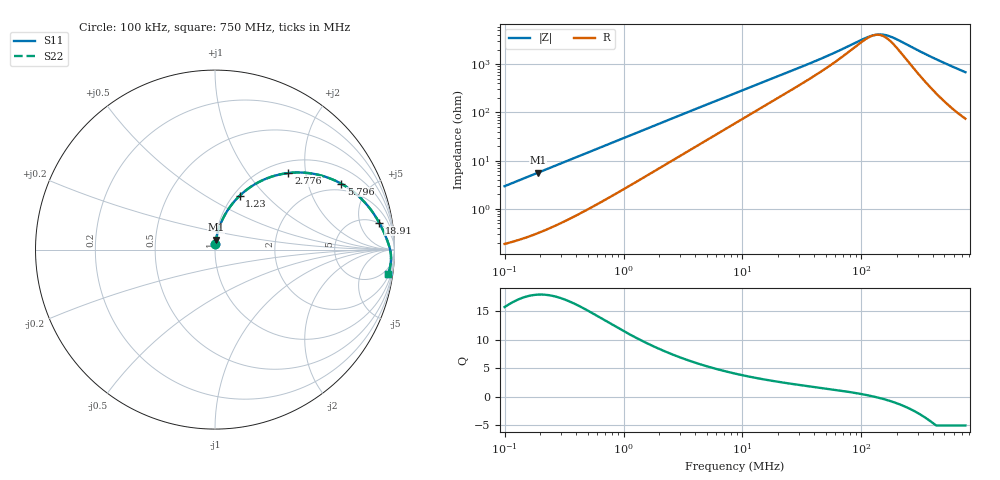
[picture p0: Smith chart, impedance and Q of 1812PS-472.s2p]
# MHz S MA R 50
!Freq  MagS11  AngS11  MagS21  AngS21  MagS12  AngS12  MagS22  AngS22
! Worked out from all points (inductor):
!   801 points, 100 kHz to 750 MHz, reference 50 ohm
!   read as one part in series: L = 4.69 uH near 104.6 kHz
!   highest Q = 17.9 at 191 kHz (marker M1), where L = 4.69 uH
!   self-resonance near 130 MHz
!   S11 on the Smith chart (normalised r, x): 100 kHz: 1.00, +0.06; 1.23 MHz: 1.07, +0.72; 2.776 MHz: 1.22, +1.61; 5.796 MHz: 1.66, +3.29; 18.91 MHz: 5, +10; 750 MHz: 2, -14
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0.1  0.02949 84.7  0.9977 -1.7  0.9977 -1.7  0.02949 84.7
0.1909598  0.0561 83.6  0.9953 -3.2  0.9953 -3.2  0.0561 83.6
0.4457309  0.1292 78.9  0.9834 -7.4  0.9834 -7.4  0.1292 78.9
0.7872414  0.2219 72.7  0.9579 -12.8  0.9579 -12.8  0.2219 72.7
1.229875  0.33 65.4  0.9132 -19.2  0.9132 -19.2  0.33 65.4
1.554466  0.3994 60.5  0.8756 -23.4  0.8756 -23.4  0.3994 60.5
1.964725  0.4754 55.1  0.8257 -28.2  0.8257 -28.2  0.4754 55.1
2.776261  0.5913 46.2  0.7287 -35.8  0.7287 -35.8  0.5913 46.2
3.923006  0.698 37.1  0.611 -43.5  0.611 -43.5  0.698 37.1
5.796327  0.7932 27.6  0.4724 -51.0  0.4724 -51.0  0.7932 27.6
8.660254  0.8597 19.6  0.3452 -56.6  0.3452 -56.6  0.8597 19.6
12.37465  0.8978 14.1  0.2543 -59.4  0.2543 -59.4  0.8978 14.1
18.90595  0.9266 9.4  0.1735 -60.4  0.1735 -60.4  0.9266 9.4
38.60143  0.9538 4.4  0.08785 -56.1  0.08785 -56.1  0.9538 4.4
58.321  0.9634 2.6  0.05719 -49.0  0.05719 -49.0  0.9634 2.6
117.7568  0.9746 0.3  0.02593 -10.9  0.02593 -10.9  0.9746 0.3
130.1909  0.9757 -0.0  0.02426 0.2  0.02426 0.2  0.9757 -0.0
142.3414  0.9767 -0.3  0.02372 11.0  0.02372 11.0  0.9767 -0.3
170.1501  0.9785 -0.8  0.02556 32.3  0.02556 32.3  0.9785 -0.8
201.136  0.9799 -1.3  0.03045 48.0  0.03045 48.0  0.9799 -1.3
419.9352  0.9819 -4.3  0.07646 74.2  0.07646 74.2  0.9819 -4.3
750  0.9743 -8.2  0.1431 75.6  0.1431 75.6  0.9743 -8.2
